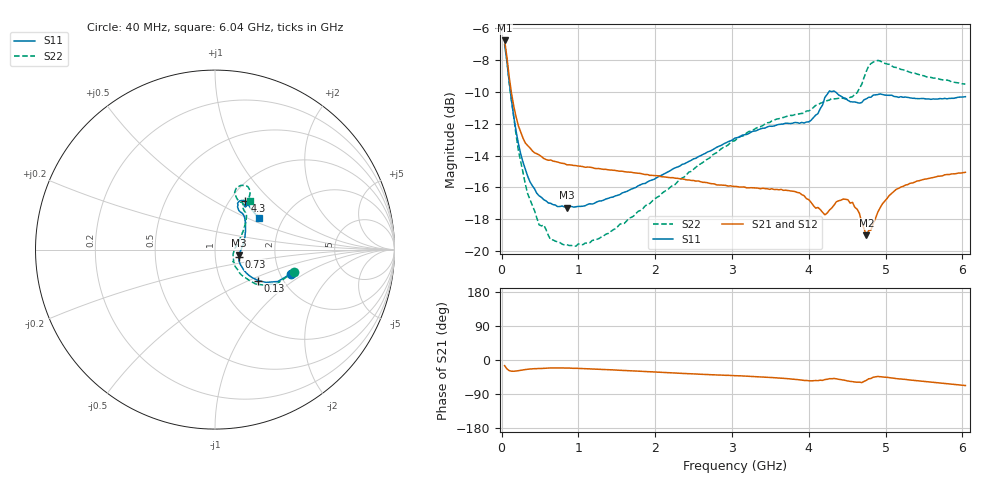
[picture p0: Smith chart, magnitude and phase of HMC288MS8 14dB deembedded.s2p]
!Hittite Microwave Corporation
!12 Elizabeth Drive
!Chelmsford, MA 01824
!Tel: 978-250-3343
!Fax: 978-250-3373
!Device: HMC288MS8, 0.7-3.7 GHz GaAs IC 3-bit Digital Attenuator in 8-lead Grounded Base surface Mount Plastic Package
!Misc:  14dB state, room
# GHZ S DB R 50.0
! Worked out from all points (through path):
!   201 points, 40 MHz to 6.04 GHz, reference 50 ohm
!   highest |S21| = -6.79 dB at 40 MHz (marker M1); lowest = -19.0 dB at 4.75 GHz (marker M2)
!   group delay of S21, straight-line fit = 20.1 ps
!   lowest |S11| = -17.3 dB at 850 MHz (marker M3), VSWR 1.32, Z = 65.2 - j4.24 ohm
!   |S11| at or under -10 dB: 115.5 MHz to 4.264 GHz (4.148 GHz wide, 189 % of centre); 4.342 GHz to end of sweep
!   |S22| runs from -19.7 to -6.8 dB; largest |S21 - S12| = 0.0026
!   S11 on the Smith chart (normalised r, x): 40 MHz: 2.29, -0.77; 130 MHz: 1.51, -0.57; 730 MHz: 1.30, -0.11; 4.3 GHz: 1.17, +0.70; 6.04 GHz: 1.52, +0.60
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0.04  -7.05 -17.6  -6.79 -15.0  -6.77 -14.9  -6.82 -15.8
0.07  -8.11 -26.8  -7.84 -23.4  -7.86 -23.2  -8.04 -28.2
0.13  -10.56 -35.6  -10.11 -29.6  -10.06 -29.3  -10.55 -40.2
0.22  -13.27 -36.7  -12.14 -28.3  -12.13 -28.2  -13.68 -43.8
0.34  -15.29 -31.9  -13.38 -24.3  -13.34 -24.6  -16.39 -40.6
0.49  -16.52 -25.7  -13.96 -22.4  -13.95 -22.3  -18.34 -34.2
0.73  -17.20 -16.9  -14.41 -21.0  -14.42 -21.1  -19.41 -20.4
0.85  -17.26 -13.4  -14.58 -21.2  -14.52 -21.4  -19.58 -15.1
1.06  -17.17 -7.3  -14.70 -22.6  -14.67 -22.6  -19.58 -6.2
2.05  -15.32 18.4  -15.28 -32.3  -15.23 -32.3  -16.55 22.7
3.04  -12.91 41.3  -15.93 -41.4  -15.88 -41.8  -13.07 40.7
3.82  -11.93 53.2  -16.25 -50.9  -16.27 -51.0  -11.43 50.7
4.06  -11.63 60.5  -17.13 -54.8  -17.09 -55.2  -10.99 56.4
4.21  -10.36 63.3  -17.71 -51.6  -17.71 -52.0  -10.60 58.2
4.3  -10.00 58.5  -17.28 -49.3  -17.30 -49.4  -10.42 58.8
4.45  -10.38 54.1  -16.73 -52.5  -16.70 -52.9  -10.42 60.9
4.57  -10.64 54.3  -16.93 -57.0  -16.95 -57.0  -10.32 65.4
4.75  -10.45 56.8  -18.99 -53.8  -18.93 -54.2  -8.72 70.9
4.87  -10.20 54.6  -17.93 -44.5  -17.89 -44.4  -8.09 64.5
5.05  -10.23 51.0  -16.50 -46.5  -16.50 -46.5  -8.29 59.6
5.32  -10.39 47.1  -15.74 -52.8  -15.70 -53.2  -8.79 57.8
6.04  -10.31 35.8  -15.05 -67.4  -15.03 -67.4  -9.53 54.3
